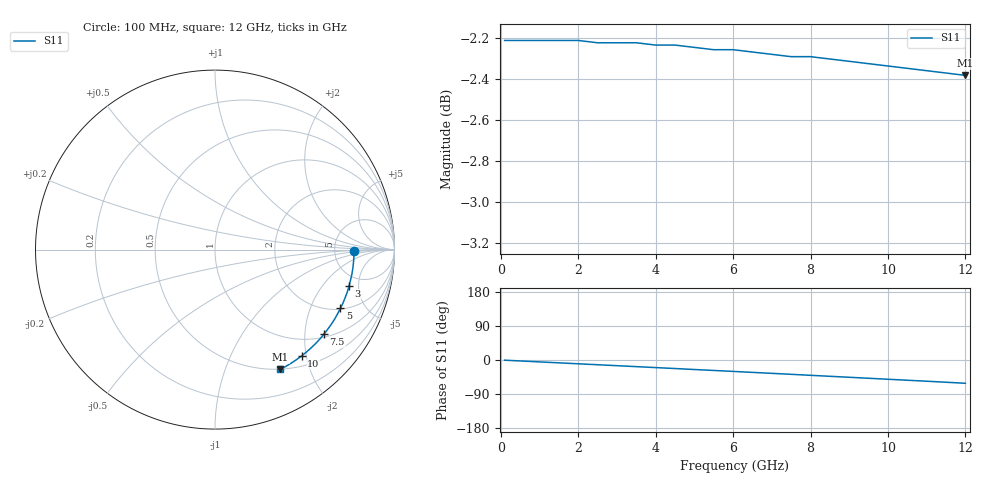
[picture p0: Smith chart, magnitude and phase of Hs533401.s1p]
!HSCH-5314 and HSCH-5334 Schottky diodes
!S-parameters at 1 mA self-bias.  Last updated 6/7/94
# ghz s ma r 50
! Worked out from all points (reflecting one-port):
!   25 points, 100 MHz to 12 GHz, reference 50 ohm
!   lowest |S11| = -2.4 dB at 12 GHz (marker M1), VSWR 7.33, Z = 24.8 - j78.5 ohm
!   phase of S11 starts at -0 deg and turns -61 deg over the sweep
!   S11 on the Smith chart (normalised r, x): 100 MHz: 7.88, -0.27; 3 GHz: 3.86, -3.86; 5 GHz: 2.04, -3.31; 7.5 GHz: 1.09, -2.50; 10 GHz: 0.67, -1.92; 12 GHz: 0.50, -1.57
0.1  0.775 -0.5
0.5  0.775 -2.5
1  0.775 -5.0
1.5  0.775 -7.5
2  0.775 -10.0
2.5  0.774 -12.5
3  0.774 -15.0
3.5  0.774 -17.5
4  0.773 -20.0
4.5  0.773 -22.5
5  0.772 -25.1
5.5  0.771 -27.6
6  0.771 -30.1
6.5  0.77 -32.7
7  0.769 -35.2
7.5  0.768 -37.8
8  0.768 -40.4
8.5  0.767 -43.0
9  0.766 -45.6
9.5  0.765 -48.2
10  0.764 -50.8
10.5  0.763 -53.4
11  0.762 -56.0
11.5  0.761 -58.7
12  0.76 -61.4
